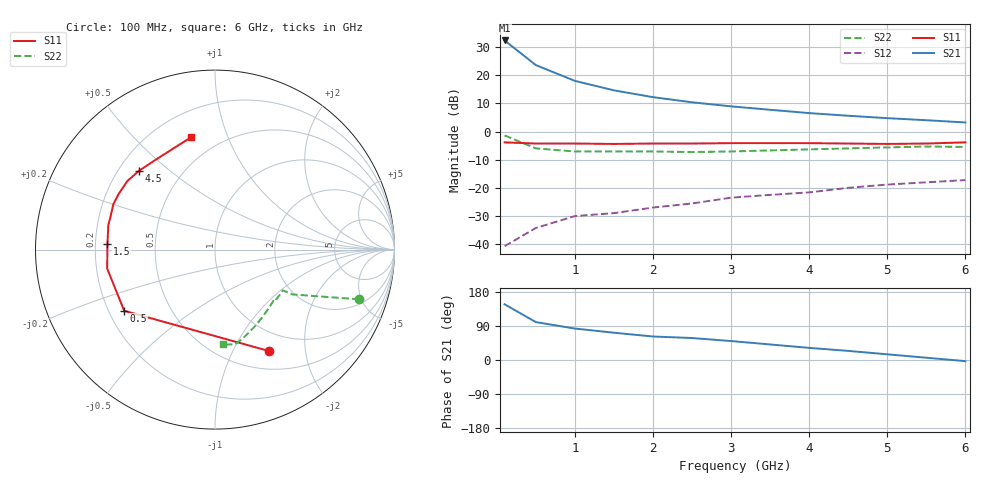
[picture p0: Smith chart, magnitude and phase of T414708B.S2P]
!AT-41470
!S-PARAMETERS at Vce=8V  Ic=25mA.  LAST UPDATED 07-21-92
# ghz s ma r 50
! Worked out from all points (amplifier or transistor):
!   13 points, 100 MHz to 6 GHz, reference 50 ohm
!   highest |S21| = 32.5 dB at 100 MHz (marker M1)
!   |S21| within 3 dB of that: start of sweep to 236.5 MHz
!   unconditionally stable (mu >= 1): 1.192 GHz to 5.047 GHz
!   at 1 GHz: K = 0.90, MSG = 24.1 dB, |S12| = -30.2 dB
!   at 3 GHz: K = 1.16, MAG = 13.9 dB, |S12| = -23.6 dB
!   at 6 GHz: K = 0.88, MSG = 10.3 dB, |S12| = -17.3 dB
!   S11 on the Smith chart (normalised r, x): 100 MHz: 0.73, -1.40; 500 MHz: 0.26, -0.29; 1.5 GHz: 0.25, +0.02; 4.5 GHz: 0.28, +0.40; 6 GHz: 0.35, +0.75
0.1  0.64 -62.0  42.11 147.0  0.009 75.0  0.85 -19.0
0.5  0.61 -146.0  15.31 100.0  0.019 47.0  0.5 -30.0
1  0.61 -170.0  8 83.0  0.031 53.0  0.44 -31.0
1.5  0.6 177.0  5.42 72.0  0.035 62.0  0.44 -34.0
2  0.61 167.0  4.1 62.0  0.044 60.0  0.44 -39.0
2.5  0.61 163.0  3.32 58.0  0.052 67.0  0.43 -39.0
3  0.62 156.0  2.81 50.0  0.066 67.0  0.44 -46.0
3.5  0.62 150.0  2.44 41.0  0.074 68.0  0.46 -55.0
4  0.62 142.0  2.13 32.0  0.082 63.0  0.48 -62.0
4.5  0.61 134.0  1.91 24.0  0.099 62.0  0.5 -68.0
5  0.6 123.0  1.73 15.0  0.113 59.0  0.52 -73.0
5.5  0.61 112.0  1.59 6.0  0.124 54.0  0.54 -78.0
6  0.64 102.0  1.45 -3.0  0.136 50.0  0.53 -85.0
